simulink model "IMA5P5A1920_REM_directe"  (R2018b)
settings: Solver=VariableStepAuto  StartTime=0.0  StopTime=5  RelTol=1e-2
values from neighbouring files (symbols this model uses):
  AB_INV = 1/AB    [Init.m]
  courant_pv = ones(PV.VT*10,1)    [Init.m]
  den = [(VEH.J/VEH.f)+(VEH.MTOT*RED.pertes*AB2)/VEH.f 1]    [Init.m]
  num = 144*(RED.pertes*AB2)/VEH.f    [Init.m]
  tension_pv = linspace(0,PV.VT,PV.VT*10)    [Init.m]
undefined symbols (not defined in the file or in its folder): ENV, irradiance_PV, MCC, RED, slselsubs, temperature_PV

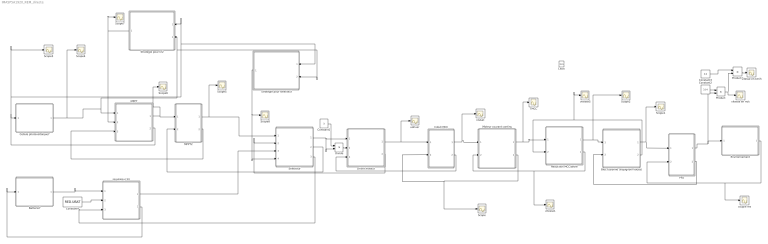
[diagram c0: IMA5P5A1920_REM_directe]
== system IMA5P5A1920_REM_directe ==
  Batterie7 : Subsystem  AncestorBlock=simulink/REM/SE
  Bloc fusionné (vispignon+roues) : Subsystem  AncestorBlock=simulink/REM/EC Elec  mask(Hacheur){}
  Cellule photovoltaïque7 : Subsystem  AncestorBlock=simulink/REM/SE
  Clock : Clock
  Constant1 : Constant  Value=3
  Constant2 : Constant  Value=3.14
  Constant3 : Constant  Value=3.6
  Constant4 : Constant  Value=RED.UBAT
  Divide : Product  Inputs=*/
  Driver moteur : Subsystem  AncestorBlock=simulink/REM/EC Elec  mask(Hacheur){}
  Environnement : Subsystem  AncestorBlock=simulink/REM/SE
  Induit MCC : Subsystem  AncestorBlock=simulink/REM/EA  mask(CM){}
  MPPT : Subsystem  AncestorBlock=simulink/REM/EC Elec  mask(Hacheur){}
  MPPT2 : Subsystem  AncestorBlock=simulink/REM/EA  mask(CM){}
  Moteur courant continu : Subsystem  AncestorBlock=simulink/REM/EC EM
  PFD : Subsystem  AncestorBlock=simulink/REM/EA  mask(CM){}
  Product : Product
  Product1 : Product
  Reduction MCC/arbre : Subsystem  AncestorBlock=simulink/REM/EC Elec  mask(Hacheur){}
  Scope{,1..8} (9 alike) : Scope
  Selecteur : Subsystem  mask(CM){}
  Strategie pour kr2 : Subsystem  AncestorBlock=simulink/SMC/Inversion EC avec mesure
  Strategie pour selecteur : Subsystem  AncestorBlock=simulink/SMC/Inversion EC avec mesure
  TMCC : Scope
  couple res : Scope
  iinduit : Scope
  regulateur 5V : Subsystem  AncestorBlock=simulink/REM/EC Elec  mask(Hacheur){}
  udriver : Scope
  vitesse en km/h : Scope
  vitesse en m/s : Scope
  vitesse1 : Scope
  vitesse5 : Scope
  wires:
  PFD/2(vvehicule) -> Bloc fusionné (vispignon+roues)/2(v_vehicule)
  Bloc fusionné (vispignon+roues)/2(Omega_arbre) -> vitesse5/1, Reduction MCC/arbre/2(Omega)
  Bloc fusionné (vispignon+roues)/1(Tred2) -> Scope1/1, PFD/1(Tred2)
  Reduction MCC/arbre/1(Tred) -> Scope2/1, Bloc fusionné (vispignon+roues)/1(Tred)
  Reduction MCC/arbre/2(OmegaMCC) -> vitesse1/1, Moteur courant continu/2(OmegaMCC)
  Driver moteur/1(Udriver) -> udriver/1, Induit MCC/1(Udriver)
  PFD/1(v_vehicule) -> Product/2, Environnement/1(V_vehicule)
  Moteur courant continu/1(TMCC) -> TMCC/1, Reduction MCC/arbre/1(TMCC)
  Moteur courant continu/2(UMCC) -> Scope/1, Induit MCC/2(UMCC)
  Induit MCC/1(I_ind) -> iinduit/1, Moteur courant continu/1(I_ind)
  Induit MCC/2(Iind) -> Driver moteur/3(Iind)
  Environnement/1(F_res) -> couple res/1, PFD/2(Fres)
  Constant2/1 -> Product/1
  Product/1 -> vitesse en m/s/1, Product1/2
  Product1/1 -> vitesse en km/h/1
  Constant3/1 -> Product1/1
  Selecteur/3(Isel2) -> regulateur 5V/3(Isel2)
  Selecteur/2(Isel1) -> MPPT2/2(Isel1)
  Batterie7/1(Ubat) -> regulateur 5V/1(Ubat)
  regulateur 5V/2(Ibat) -> Batterie7/1(Ibat)
  regulateur 5V/1(U5v) -> Selecteur/3(Ubatt)
  Constant4/1 -> regulateur 5V/2(mreg)
  MPPT/1(Imppt) -> Scope6/1, MPPT2/1(Imppt)
  MPPT2/1(Umppt) -> Scope5/1, Selecteur/1(Umppt)
  MPPT2/2(U_mppt) -> MPPT/3(Umppt)
  Driver moteur/2(Idriver) -> Selecteur/2(Idriver)
  Cellule photovoltaïque7/1(Ipv) -> Scope4/1, Strategie pour selecteur/2(Ipv), Strategie pour kr2/2(Ipv), MPPT/1(Ipv)
  Strategie pour kr2/1(mh) -> Scope7/1, MPPT/2(mh)
  MPPT/2(Uint) -> Scope3/1, Strategie pour kr2/1(Upv), Strategie pour selecteur/1(Upv), Cellule photovoltaïque7/1(Uint)
  Strategie pour selecteur/1(selecteur) -> Scope8/1, Selecteur/4(selecteur)
  Selecteur/1(Usel) -> Divide/2, Driver moteur/1(Usel)
  Divide/1 -> Driver moteur/2(reg_uP)
  Constant1/1 -> Divide/1
  Clock/1 -> ?

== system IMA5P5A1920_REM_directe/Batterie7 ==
  Ibat : Inport
  Constant : Constant  Value=9
  Scope : Scope
  Ubat : Outport  InitialOutput=0
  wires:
  Constant/1 -> Ubat/1
  Ibat/1 -> Scope/1

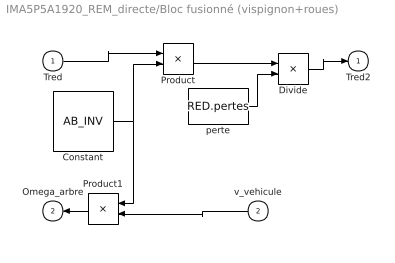
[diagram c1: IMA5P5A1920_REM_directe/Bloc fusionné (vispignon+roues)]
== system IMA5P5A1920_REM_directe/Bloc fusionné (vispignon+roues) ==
  Tred : Inport
  v_vehicule : Inport  Port=2
  Constant : Constant  Value=AB_INV
  Divide : Product  Inputs=*/
  Product : Product
  Product1 : Product
  perte : Constant  Value=RED.pertes
  Tred2 : Outport  InitialOutput=0
  Omega_arbre : Outport  Port=2  InitialOutput=0
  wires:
  Tred/1 -> Product/1
  Product/1 -> Divide/1
  Product1/1 -> Omega_arbre/1
  v_vehicule/1 -> Product1/2
  Constant/1 -> Product1/1, Product/2
  perte/1 -> Divide/2
  Divide/1 -> Tred2/1

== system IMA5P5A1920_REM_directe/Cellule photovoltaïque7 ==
  Uint : Inport
  Gain : Gain
  Look-Up Table (n-D) : Lookup_n-D  NumberOfTableDimensions=1  BreakpointsForDimension1=tension_pv  BreakpointsForDimension2=irradiance_PV  BreakpointsForDimension3=temperature_PV  BreakpointsForDimension5=slselsubs({[1:3], [1:3], [1:3], [1:3], [1:3], [1:3], [1:3], [1:3], [1:3], [1:3], [1:3], [1:3], [1:3], [1:3], [1:3], [1:3], [1:3], [1:3], [1:3], [1:3], [1:3], [1:3], [1:3], [1:3], [1:3], [1:3]}, 1)  BreakpointsForDimension6=slselsubs({[1:3], [1:3], [1:3], [1:3], [1:3], [1:3], [1:3], [1:3], [1:3], [1:3], [1:3], [1:3], [1:3], [1:3], [1:3], [1:3], [1:3], [1:3], [1:3], [1:3], [1:3], [1:3], [1:3], [1:3], [1:3], [1:3]}, 2)  BreakpointsForDimension7=slselsubs({[1:3], [1:3], [1:3], [1:3], [1:3], [1:3], [1:3], [1:3], [1:3], [1:3], [1:3], [1:3], [1:3], [1:3], [1:3], [1:3], [1:3], [1:3], [1:3], [1:3], [1:3], [1:3], [1:3], [1:3], [1:3], [1:3]}, 3)  BreakpointsForDimension8=slselsubs({[1:3], [1:3], [1:3], [1:3], [1:3], [1:3], [1:3], [1:3], [1:3], [1:3], [1:3], [1:3], [1:3], [1:3], [1:3], [1:3], [1:3], [1:3], [1:3], [1:3], [1:3], [1:3], [1:3], [1:3], [1:3], [1:3]}, 4)  BreakpointsForDimension9=slselsubs({[1:3], [1:3], [1:3], [1:3], [1:3], [1:3], [1:3], [1:3], [1:3], [1:3], [1:3], [1:3], [1:3], [1:3], [1:3], [1:3], [1:3], [1:3], [1:3], [1:3], [1:3], [1:3], [1:3], [1:3], [1:3], [1:3]}, 5)  BreakpointsForDimension10=slselsubs({[1:3], [1:3], [1:3], [1:3], [1:3], [1:3], [1:3], [1:3], [1:3], [1:3], [1:3], [1:3], [1:3], [1:3], [1:3], [1:3], [1:3], [1:3], [1:3], [1:3], [1:3], [1:3], [1:3], [1:3], [1:3], [1:3]}, 6)  BreakpointsForDimension11=slselsubs({[1:3], [1:3], [1:3], [1:3], [1:3], [1:3], [1:3], [1:3], [1:3], [1:3], [1:3], [1:3], [1:3], [1:3], [1:3], [1:3], [1:3], [1:3], [1:3], [1:3], [1:3], [1:3], [1:3], [1:3], [1:3], [1:3]}, 7)  BreakpointsForDimension12=slselsubs({[1:3], [1:3], [1:3], [1:3], [1:3], [1:3], [1:3], [1:3], [1:3], [1:3], [1:3], [1:3], [1:3], [1:3], [1:3], [1:3], [1:3], [1:3], [1:3], [1:3], [1:3], [1:3], [1:3], [1:3], [1:3], [1:3]}, 8)  BreakpointsForDimension13=slselsubs({[1:3], [1:3], [1:3], [1:3], [1:3], [1:3], [1:3], [1:3], [1:3], [1:3], [1:3], [1:3], [1:3], [1:3], [1:3], [1:3], [1:3], [1:3], [1:3], [1:3], [1:3], [1:3], [1:3], [1:3], [1:3], [1:3]}, 9)  BreakpointsForDimension14=slselsubs({[1:3], [1:3], [1:3], [1:3], [1:3], [1:3], [1:3], [1:3], [1:3], [1:3], [1:3], [1:3], [1:3], [1:3], [1:3], [1:3], [1:3], [1:3], [1:3], [1:3], [1:3], [1:3], [1:3], [1:3], [1:3], [1:3]}, 10)  BreakpointsForDimension15=slselsubs({[1:3], [1:3], [1:3], [1:3], [1:3], [1:3], [1:3], [1:3], [1:3], [1:3], [1:3], [1:3], [1:3], [1:3], [1:3], [1:3], [1:3], [1:3], [1:3], [1:3], [1:3], [1:3], [1:3], [1:3], [1:3], [1:3]}, 11)  BreakpointsForDimension16=slselsubs({[1:3], [1:3], [1:3], [1:3], [1:3], [1:3], [1:3], [1:3], [1:3], [1:3], [1:3], [1:3], [1:3], [1:3], [1:3], [1:3], [1:3], [1:3], [1:3], [1:3], [1:3], [1:3], [1:3], [1:3], [1:3], [1:3]}, 12)  BreakpointsForDimension17=slselsubs({[1:3], [1:3], [1:3], [1:3], [1:3], [1:3], [1:3], [1:3], [1:3], [1:3], [1:3], [1:3], [1:3], [1:3], [1:3], [1:3], [1:3], [1:3], [1:3], [1:3], [1:3], [1:3], [1:3], [1:3], [1:3], [1:3]}, 13)  BreakpointsForDimension18=slselsubs({[1:3], [1:3], [1:3], [1:3], [1:3], [1:3], [1:3], [1:3], [1:3], [1:3], [1:3], [1:3], [1:3], [1:3], [1:3], [1:3], [1:3], [1:3], [1:3], [1:3], [1:3], [1:3], [1:3], [1:3], [1:3], [1:3]}, 14)  BreakpointsForDimension19=slselsubs({[1:3], [1:3], [1:3], [1:3], [1:3], [1:3], [1:3], [1:3], [1:3], [1:3], [1:3], [1:3], [1:3], [1:3], [1:3], [1:3], [1:3], [1:3], [1:3], [1:3], [1:3], [1:3], [1:3], [1:3], [1:3], [1:3]}, 15)  BreakpointsForDimension20=slselsubs({[1:3], [1:3], [1:3], [1:3], [1:3], [1:3], [1:3], [1:3], [1:3], [1:3], [1:3], [1:3], [1:3], [1:3], [1:3], [1:3], [1:3], [1:3], [1:3], [1:3], [1:3], [1:3], [1:3], [1:3], [1:3], [1:3]}, 16)  BreakpointsForDimension21=slselsubs({[1:3], [1:3], [1:3], [1:3], [1:3], [1:3], [1:3], [1:3], [1:3], [1:3], [1:3], [1:3], [1:3], [1:3], [1:3], [1:3], [1:3], [1:3], [1:3], [1:3], [1:3], [1:3], [1:3], [1:3], [1:3], [1:3]}, 17)  BreakpointsForDimension22=slselsubs({[1:3], [1:3], [1:3], [1:3], [1:3], [1:3], [1:3], [1:3], [1:3], [1:3], [1:3], [1:3], [1:3], [1:3], [1:3], [1:3], [1:3], [1:3], [1:3], [1:3], [1:3], [1:3], [1:3], [1:3], [1:3], [1:3]}, 18)  BreakpointsForDimension23=slselsubs({[1:3], [1:3], [1:3], [1:3], [1:3], [1:3], [1:3], [1:3], [1:3], [1:3], [1:3], [1:3], [1:3], [1:3], [1:3], [1:3], [1:3], [1:3], [1:3], [1:3], [1:3], [1:3], [1:3], [1:3], [1:3], [1:3]}, 19)  BreakpointsForDimension24=slselsubs({[1:3], [1:3], [1:3], [1:3], [1:3], [1:3], [1:3], [1:3], [1:3], [1:3], [1:3], [1:3], [1:3], [1:3], [1:3], [1:3], [1:3], [1:3], [1:3], [1:3], [1:3], [1:3], [1:3], [1:3], [1:3], [1:3]}, 20)  BreakpointsForDimension25=slselsubs({[1:3], [1:3], [1:3], [1:3], [1:3], [1:3], [1:3], [1:3], [1:3], [1:3], [1:3], [1:3], [1:3], [1:3], [1:3], [1:3], [1:3], [1:3], [1:3], [1:3], [1:3], [1:3], [1:3], [1:3], [1:3], [1:3]}, 21)  BreakpointsForDimension26=slselsubs({[1:3], [1:3], [1:3], [1:3], [1:3], [1:3], [1:3], [1:3], [1:3], [1:3], [1:3], [1:3], [1:3], [1:3], [1:3], [1:3], [1:3], [1:3], [1:3], [1:3], [1:3], [1:3], [1:3], [1:3], [1:3], [1:3]}, 22)  BreakpointsForDimension27=slselsubs({[1:3], [1:3], [1:3], [1:3], [1:3], [1:3], [1:3], [1:3], [1:3], [1:3], [1:3], [1:3], [1:3], [1:3], [1:3], [1:3], [1:3], [1:3], [1:3], [1:3], [1:3], [1:3], [1:3], [1:3], [1:3], [1:3]}, 23)  BreakpointsForDimension28=slselsubs({[1:3], [1:3], [1:3], [1:3], [1:3], [1:3], [1:3], [1:3], [1:3], [1:3], [1:3], [1:3], [1:3], [1:3], [1:3], [1:3], [1:3], [1:3], [1:3], [1:3], [1:3], [1:3], [1:3], [1:3], [1:3], [1:3]}, 24)  BreakpointsForDimension29=slselsubs({[1:3], [1:3], [1:3], [1:3], [1:3], [1:3], [1:3], [1:3], [1:3], [1:3], [1:3], [1:3], [1:3], [1:3], [1:3], [1:3], [1:3], [1:3], [1:3], [1:3], [1:3], [1:3], [1:3], [1:3], [1:3], [1:3]}, 25)  BreakpointsForDimension30=slselsubs({[1:3], [1:3], [1:3], [1:3], [1:3], [1:3], [1:3], [1:3], [1:3], [1:3], [1:3], [1:3], [1:3], [1:3], [1:3], [1:3], [1:3], [1:3], [1:3], [1:3], [1:3], [1:3], [1:3], [1:3], [1:3], [1:3]}, 26)  Table=courant_pv  InterpMethod=Cubic spline  ExtrapMethod=Cubic spline  InternalRulePriority=Speed  RndMeth=Simplest
  limitation : Saturate  UpperLimit=inf  LowerLimit=0
  Ipv : Outport  InitialOutput=0
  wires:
  limitation/1 -> Ipv/1
  Uint/1 -> Look-Up Table (n-D)/1
  Gain/1 -> limitation/1
  Look-Up Table (n-D)/1 -> Gain/1

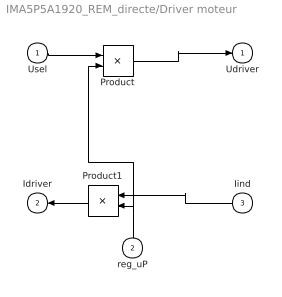
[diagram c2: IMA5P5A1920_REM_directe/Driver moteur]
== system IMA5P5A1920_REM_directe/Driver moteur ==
  Usel : Inport
  reg_uP : Inport  Port=2
  Iind : Inport  Port=3
  Product : Product
  Product1 : Product
  Udriver : Outport  InitialOutput=0
  Idriver : Outport  Port=2  InitialOutput=0
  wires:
  reg_uP/1 -> Product1/2, Product/2
  Usel/1 -> Product/1
  Product/1 -> Udriver/1
  Iind/1 -> Product1/1
  Product1/1 -> Idriver/1

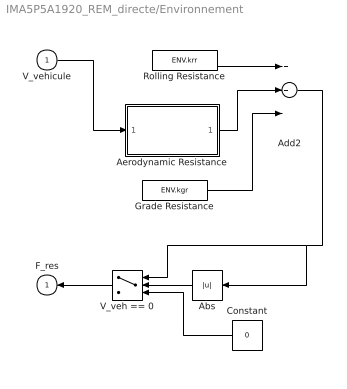
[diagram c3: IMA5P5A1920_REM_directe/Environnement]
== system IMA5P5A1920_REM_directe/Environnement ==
  V_vehicule : Inport
  Abs : Abs
  Add2 : Sum  Inputs=3
  Aerodynamic Resistance : Subsystem
  Constant : Constant  Value=0
  Grade Resistance : Constant  Value=ENV.kgr
  Rolling Resistance : Constant  Value=ENV.krr
  V_veh == 0 : Switch  Threshold=0.1
  F_res : Outport  InitialOutput=0
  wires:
  Add2/1 -> Abs/1, V_veh == 0/1
  Abs/1 -> V_veh == 0/2
  Rolling Resistance/1 -> Add2/1
  Aerodynamic Resistance/1(F_ar) -> Add2/2
  V_veh == 0/1 -> F_res/1
  Grade Resistance/1 -> Add2/3
  V_vehicule/1 -> Aerodynamic Resistance/1(V_veh)
  Constant/1 -> V_veh == 0/3

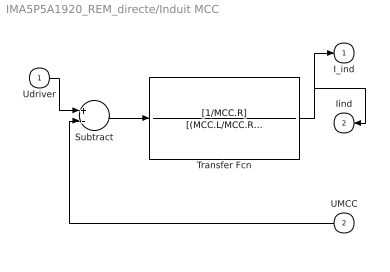
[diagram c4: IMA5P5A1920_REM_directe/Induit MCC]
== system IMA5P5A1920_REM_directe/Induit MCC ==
  Udriver : Inport
  UMCC : Inport  Port=2
  Subtract : Sum  Inputs=+-
  Transfer Fcn : TransferFcn  Numerator=[1/MCC.R]  Denominator=[(MCC.L/MCC.R) 1]
  I_ind : Outport  InitialOutput=0
  Iind : Outport  Port=2  InitialOutput=0
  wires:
  Udriver/1 -> Subtract/1
  UMCC/1 -> Subtract/2
  Transfer Fcn/1 -> Iind/1, I_ind/1
  Subtract/1 -> Transfer Fcn/1

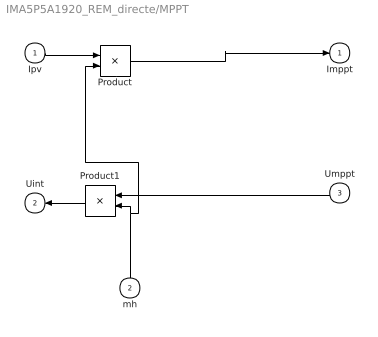
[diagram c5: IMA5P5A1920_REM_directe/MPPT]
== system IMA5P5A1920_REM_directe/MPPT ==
  Ipv : Inport
  mh : Inport  Port=2
  Umppt : Inport  Port=3
  Product : Product
  Product1 : Product
  Imppt : Outport  InitialOutput=0
  Uint : Outport  Port=2  InitialOutput=0
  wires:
  mh/1 -> Product/2, Product1/2
  Ipv/1 -> Product/1
  Umppt/1 -> Product1/1
  Product1/1 -> Uint/1
  Product/1 -> Imppt/1

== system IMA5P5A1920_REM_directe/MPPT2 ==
  Imppt : Inport
  Isel1 : Inport  Port=2
  Subtract : Sum  Inputs=+-
  Transfer Fcn : TransferFcn  Numerator=10  Denominator=[0.3 1]
  Umppt : Outport  InitialOutput=0
  U_mppt : Outport  Port=2  InitialOutput=0
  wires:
  Imppt/1 -> Subtract/1
  Isel1/1 -> Subtract/2
  Subtract/1 -> Transfer Fcn/1
  Transfer Fcn/1 -> U_mppt/1, Umppt/1

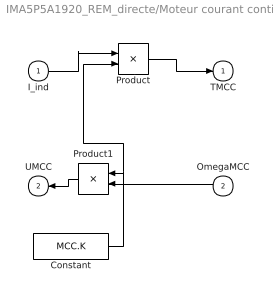
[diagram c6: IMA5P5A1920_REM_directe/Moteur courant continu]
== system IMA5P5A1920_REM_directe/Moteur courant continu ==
  I_ind : Inport
  OmegaMCC : Inport  Port=2
  Constant : Constant  Value=MCC.K
  Product : Product
  Product1 : Product
  TMCC : Outport  InitialOutput=0
  UMCC : Outport  Port=2  InitialOutput=0
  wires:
  I_ind/1 -> Product/1
  Constant/1 -> Product1/1, Product/2
  Product/1 -> TMCC/1
  OmegaMCC/1 -> Product1/2
  Product1/1 -> UMCC/1

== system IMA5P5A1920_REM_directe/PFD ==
  Tred2 : Inport
  Fres : Inport  Port=2
  Subtract : Sum  Inputs=+-
  Transfer Fcn : TransferFcn  Numerator=num  Denominator=den
  v_vehicule : Outport  InitialOutput=0
  vvehicule : Outport  Port=2  InitialOutput=0
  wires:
  Fres/1 -> Subtract/2
  Tred2/1 -> Subtract/1
  Transfer Fcn/1 -> vvehicule/1, v_vehicule/1
  Subtract/1 -> Transfer Fcn/1

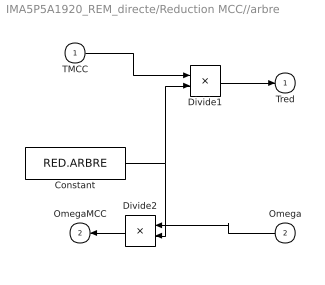
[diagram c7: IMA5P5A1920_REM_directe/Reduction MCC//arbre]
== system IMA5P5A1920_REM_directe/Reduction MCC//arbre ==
  TMCC : Inport
  Omega : Inport  Port=2
  Constant : Constant  Value=RED.ARBRE
  Divide1 : Product  Inputs=*/
  Divide2 : Product  Inputs=*/
  Tred : Outport  InitialOutput=0
  OmegaMCC : Outport  Port=2  InitialOutput=0
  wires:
  TMCC/1 -> Divide1/1
  Divide1/1 -> Tred/1
  Divide2/1 -> OmegaMCC/1
  Constant/1 -> Divide2/2, Divide1/2
  Omega/1 -> Divide2/1

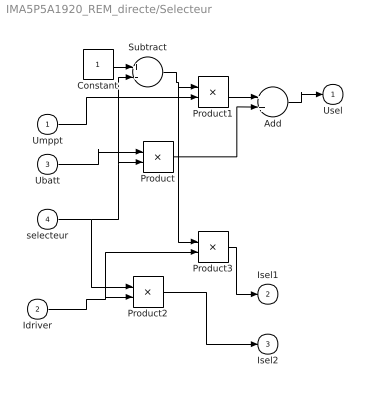
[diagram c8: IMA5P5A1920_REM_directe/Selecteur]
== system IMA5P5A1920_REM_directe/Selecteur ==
  Umppt : Inport
  Idriver : Inport  Port=2
  Ubatt : Inport  Port=3
  selecteur : Inport  Port=4
  Add : Sum
  Constant : Constant
  Product{,1..3} (4 alike) : Product
  Subtract : Sum  Inputs=+-
  Usel : Outport  InitialOutput=0
  Isel1 : Outport  Port=2  InitialOutput=0
  Isel2 : Outport  Port=3  InitialOutput=0
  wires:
  Ubatt/1 -> Product/1
  selecteur/1 -> Product2/1, Subtract/2, Product/2
  Constant/1 -> Subtract/1
  Umppt/1 -> Product1/2
  Subtract/1 -> Product3/1, Product1/1
  Product/1 -> Add/2
  Product1/1 -> Add/1
  Add/1 -> Usel/1
  Idriver/1 -> Product3/2, Product2/2
  Product2/1 -> Isel2/1
  Product3/1 -> Isel1/1

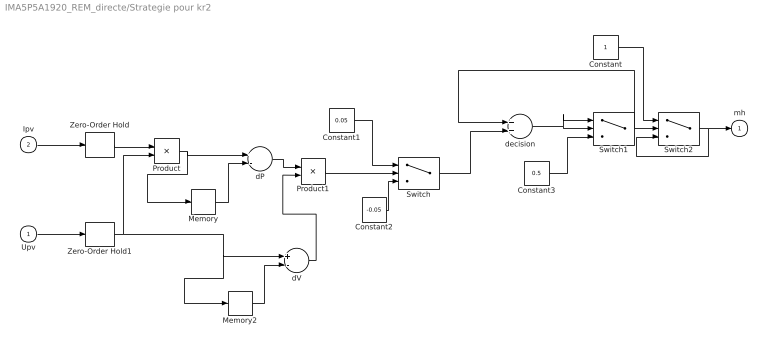
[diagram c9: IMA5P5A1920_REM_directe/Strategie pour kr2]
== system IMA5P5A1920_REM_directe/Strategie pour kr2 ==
  Upv : Inport
  Ipv : Inport  Port=2
  Constant : Constant
  Constant1 : Constant  Value=0.05
  Constant2 : Constant  Value=-0.05
  Constant3 : Constant  Value=0.5
  Memory : Memory  InheritSampleTime=on  LinearizeMemory=on  LinearizeAsDelay=on
  Memory2 : Memory  InheritSampleTime=on  LinearizeMemory=on  LinearizeAsDelay=on
  Product : Product
  Product1 : Product
  Switch : Switch  Criteria=u2 > Threshold
  Switch1 : Switch  Criteria=u2 > Threshold
  Switch2 : Switch  Criteria=u2 > Threshold  Threshold=1
  Zero-Order Hold : ZeroOrderHold  SampleTime=-1
  Zero-Order Hold1 : ZeroOrderHold  SampleTime=-1
  dP : Sum  Inputs=+-
  dV : Sum  Inputs=+-
  decision : Sum
  mh : Outport  InitialOutput=0
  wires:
  Zero-Order Hold/1 -> Product/1
  Memory/1 -> dP/2
  Ipv/1 -> Zero-Order Hold/1
  Upv/1 -> Zero-Order Hold1/1
  Switch1/1 -> Switch2/2, decision/1
  Zero-Order Hold1/1 -> Memory2/1, dV/1, Product/2
  Memory2/1 -> dV/2
  dP/1 -> Product1/1
  dV/1 -> Product1/2
  Product1/1 -> Switch/2
  Constant1/1 -> Switch/1
  Constant2/1 -> Switch/3
  Switch/1 -> decision/2
  decision/1 -> Switch1/1, Switch1/2
  Constant3/1 -> Switch1/3
  Product/1 -> Memory/1, dP/1
  Constant/1 -> Switch2/1
  Switch2/1 -> Switch2/3, mh/1

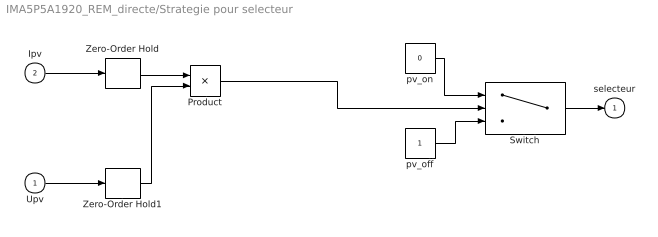
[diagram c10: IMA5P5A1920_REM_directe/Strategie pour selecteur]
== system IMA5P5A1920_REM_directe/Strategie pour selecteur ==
  Upv : Inport
  Ipv : Inport  Port=2
  Product : Product
  Switch : Switch  Threshold=3
  Zero-Order Hold : ZeroOrderHold  SampleTime=-1
  Zero-Order Hold1 : ZeroOrderHold  SampleTime=-1
  pv_off : Constant
  pv_on : Constant  Value=0
  selecteur : Outport  InitialOutput=0
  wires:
  Zero-Order Hold/1 -> Product/1
  Ipv/1 -> Zero-Order Hold/1
  Upv/1 -> Zero-Order Hold1/1
  Zero-Order Hold1/1 -> Product/2
  Product/1 -> Switch/2
  pv_on/1 -> Switch/1
  pv_off/1 -> Switch/3
  Switch/1 -> selecteur/1

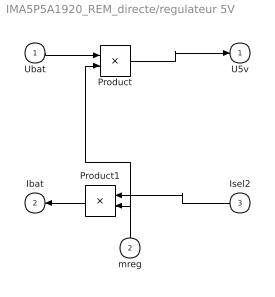
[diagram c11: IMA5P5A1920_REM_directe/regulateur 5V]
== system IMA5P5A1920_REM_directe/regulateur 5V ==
  Ubat : Inport
  mreg : Inport  Port=2
  Isel2 : Inport  Port=3
  Product : Product
  Product1 : Product
  U5v : Outport  InitialOutput=0
  Ibat : Outport  Port=2  InitialOutput=0
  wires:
  mreg/1 -> Product1/2, Product/2
  Ubat/1 -> Product/1
  Product/1 -> U5v/1
  Isel2/1 -> Product1/1
  Product1/1 -> Ibat/1

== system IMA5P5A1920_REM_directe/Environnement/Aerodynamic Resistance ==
  V_veh : Inport
  Add1 : Sum
  Constant2 : Constant  Value=ENV.Vwind
  Gain3 : Gain  Gain=ENV.kaero
  Product : Product
  F_ar : Outport  InitialOutput=0
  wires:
  Gain3/1 -> F_ar/1
  Product/1 -> Gain3/1
  Add1/1 -> Product/1, Product/2
  Constant2/1 -> Add1/2
  V_veh/1 -> Add1/1
